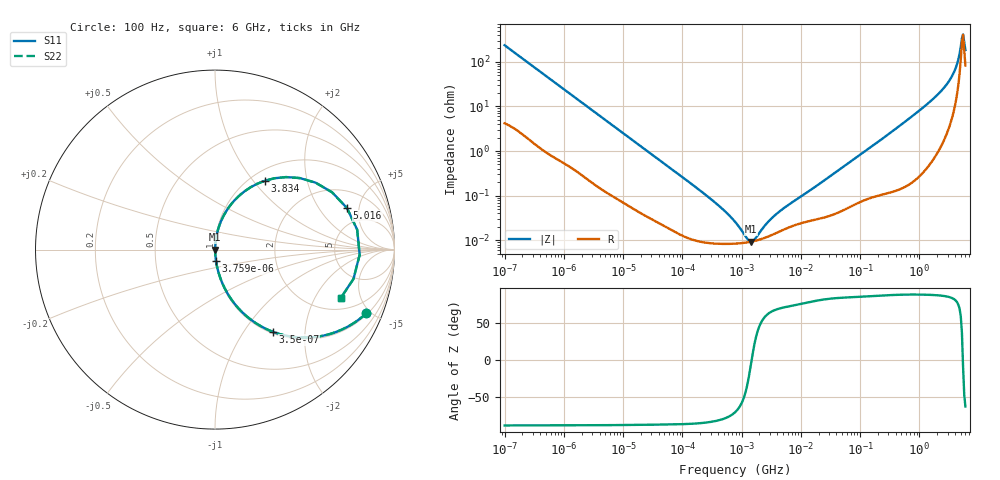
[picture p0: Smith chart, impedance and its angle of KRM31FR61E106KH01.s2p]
!Murata Part Number: KRM31FR61E106KH01
!These Parameters are Measured in Series Mode Connection
!Data Generated on Jan 08, 2026
!  o--ll--o
!Port1  Port2
!  o------o
!Operation Temp=25[degC], DC Bias Voltage=0[V]
!Freq. Start=100[Hz] Stop=6[GHz] 401[Steps]
# Hz S RI R 50
!Freq.(Hz) S11(Real) S11(Imag) S21(Real) S21(Imag) S12(Real) S12(Imag) S22(Real) S22(Imag)
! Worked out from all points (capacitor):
!   401 points, 100 Hz to 6 GHz, reference 50 ohm
!   read as one part in series: C = 6.71 uF near 109 Hz
!   lowest |Z| = 9.3 mohm at 1.45 MHz (marker M1)
!   series resonance near 1.483 MHz, so ESL is about 1.7 nH
!   S11 on the Smith chart (normalised r, x): 100 Hz: 1.08, -4.72; 350 Hz: 1.03, -1.37; 3.759 kHz: 1.00, -0.13; 3.834 GHz: 1.16, +1.15; 5.016 GHz: 3.28, +3.74; 6 GHz: 2.66, -3.31
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100  0.8434 -0.3546  0.1566 0.3546  0.1566 0.3546  0.8434 -0.3546
205  0.5748 -0.4845  0.4252 0.4845  0.4252 0.4845  0.5748 -0.4845
350  0.3233 -0.4583  0.6767 0.4583  0.6767 0.4583  0.3233 -0.4583
750  0.0994 -0.289  0.9006 0.289  0.9006 0.289  0.0994 -0.289
2008  0.0175 -0.12  0.9825 0.12  0.9825 0.12  0.0175 -0.12
3759  0.00588 -0.0655  0.9941 0.0655  0.9941 0.0655  0.00588 -0.0655
40335  0.000283 -0.00639  0.9997 0.00639  0.9997 0.00639  0.000283 -0.00639
316350  8.57e-05 -0.000796  0.9999 0.000796  0.9999 0.000796  8.57e-05 -0.000796
774597  8.39e-05 -0.000247  0.9999 0.000247  0.9999 0.000247  8.39e-05 -0.000247
1212075  8.9e-05 -7.13e-05  0.9999 7.13e-05  0.9999 7.13e-05  8.9e-05 -7.13e-05
1449809  9.27e-05 -7.8e-06  0.9999 7.8e-06  0.9999 7.8e-06  9.27e-05 -7.8e-06
1734173  9.79e-05 5.45e-05  0.9999 -5.45e-05  0.9999 -5.45e-05  9.79e-05 5.45e-05
3882480  0.000146 0.000361  0.9999 -0.000361  0.9999 -0.000361  0.000146 0.000361
1.555665e7  0.00028 0.00139  0.9997 -0.00139  0.9997 -0.00139  0.00028 0.00139
3.124326e8  0.00177 0.0246  0.9982 -0.0246  0.9982 -0.0246  0.00177 0.0246
2.142435e9  0.0463 0.1853  0.9537 -0.1853  0.9537 -0.1853  0.0463 0.1853
3.065283e9  0.1263 0.2923  0.8737 -0.2923  0.8737 -0.2923  0.1263 0.2923
3.8344e9  0.2785 0.3838  0.7215 -0.3838  0.7215 -0.3838  0.2785 0.3838
4.385646e9  0.4731 0.3984  0.5269 -0.3984  0.5269 -0.3984  0.4731 0.3984
5.016141e9  0.7353 0.2315  0.2647 -0.2315  0.2647 -0.2315  0.7353 0.2315
5.486059e9  0.806 -0.0289  0.194 0.0289  0.194 0.0289  0.806 -0.0289
6e9  0.6992 -0.2719  0.3008 0.2719  0.3008 0.2719  0.6992 -0.2719
